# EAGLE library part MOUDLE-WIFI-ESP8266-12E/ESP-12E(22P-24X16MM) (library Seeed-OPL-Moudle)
317060015
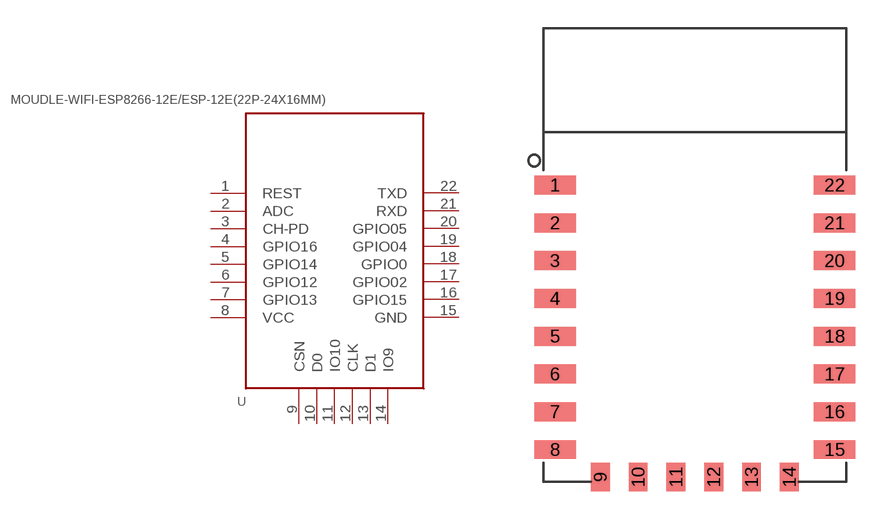
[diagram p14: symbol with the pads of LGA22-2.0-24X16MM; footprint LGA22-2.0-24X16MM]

Designator prefix U

## MOUDLE-WIFI-ESP8266-12E/ESP-12E(22P-24X16MM) (MPN: ESP8266-12E/ESP-12E; VALUE: ESP8266-12E/ESP-12E)  [LGA22-2.0-24X16MM]
1  REST
2  ADC
3  CH-PD
4  GPIO16
5  GPIO14
6  GPIO12
7  GPIO13
8  VCC
9  CSN
10  D0
11  IO10
12  CLK
13  D1
14  IO9
15  GND
16  GPIO15
17  GPIO02
18  GPIO0
19  GPIO04
20  GPIO05
21  RXD
22  TXD

## Footprint LGA22-2.0-24X16MM (pad centres in mm)
smd 2.2 x 1: 1 -7.4,3.7; 2 -7.4,1.7; 3 -7.4,-0.3; 4 -7.4,-2.3; 5 -7.4,-4.3; 6 -7.4,-6.3; 7 -7.4,-8.3; 8 -7.4,-10.3; 15 7.4,-10.3; 16 7.4,-8.3; 17 7.4,-6.3; 18 7.4,-4.3; 19 7.4,-2.3; 20 7.4,-0.3; 21 7.4,1.7; 22 7.4,3.7
smd 1 x 1.5: 9 -5,-11.75; 10 -3,-11.75; 11 -1,-11.75; 12 1,-11.75; 13 3,-11.75; 14 5,-11.75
